(* Logix 5000 AddOnInstructionDefinition export Bronkhorst_FF_Extended_REAL_Input; software revision 37.00 *)

ADD_ON_INSTRUCTION Bronkhorst_FF_Extended_REAL_Input   (* revision 1.0, vendor Bronkhorst High-Tech B.V. *)
// Extract data from the FLEXI-FLOW Extended REAL input connection (in to controller from device)
VAR_IN_OUT
   DataIn : SINT[30]; {required}
END_VAR
VAR_OUTPUT
   Status : USINT; {visible}
   Measure : REAL; {visible}
   Setpoint : REAL; {visible}
   Override : USINT; {visible}
   Actuator : REAL; {visible}
   Pressure_Inlet : REAL; {visible}
   Pressure_Inlet_Setpoint : REAL; {visible}
   Pressure_Outlet : REAL; {visible}
   Pressure_Outlet_Setpoint : REAL; {visible}
END_VAR

ROUTINE Logic   (* structured text *)
   Status := DataIn[0];
   COP(DataIn[1], Measure, 1);
   COP(DataIn[5], Setpoint, 1);
   Override := DataIn[9];
   COP(DataIn[10], Actuator, 1);
   COP(DataIn[14], Pressure_Inlet, 1);
   COP(DataIn[18], Pressure_Inlet_Setpoint, 1);
   COP(DataIn[22], Pressure_Outlet, 1);
   COP(DataIn[26], Pressure_Outlet_Setpoint, 1);
END_ROUTINE
END_ADD_ON_INSTRUCTION

ADD_ON_INSTRUCTION Bronkhorst_FF_Extended_REAL_Output   (* revision 1.0, vendor Bronkhorst High-Tech B.V. *)
// Fill data for the FLEXI-FLOW Extended REAL output connection (out from controller to device)
VAR_IN_OUT
   DataOut : SINT[13]; {required}
END_VAR
VAR_INPUT
   Override : USINT; {visible}
   Setpoint : REAL; {visible}
   Pressure_Inlet_Setpoint : REAL; {visible}
   Pressure_Outlet_Setpoint : REAL; {visible}
END_VAR

ROUTINE Logic   (* structured text *)
   DataOut[0] := Override;
   COP(Setpoint, DataOut[1], 4);
   COP(Pressure_Inlet_Setpoint, DataOut[5], 4);
   COP(Pressure_Outlet_Setpoint, DataOut[9], 4);
END_ROUTINE
END_ADD_ON_INSTRUCTION
